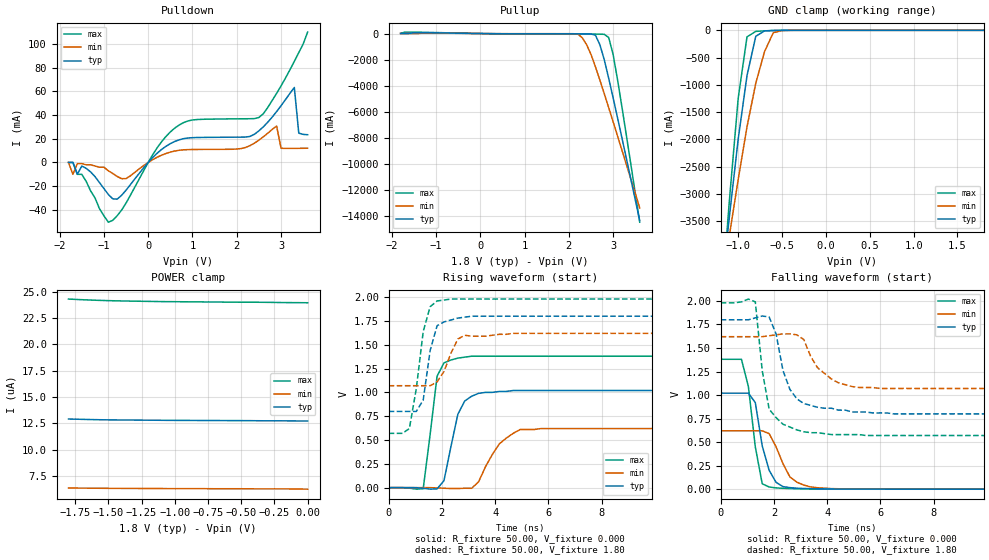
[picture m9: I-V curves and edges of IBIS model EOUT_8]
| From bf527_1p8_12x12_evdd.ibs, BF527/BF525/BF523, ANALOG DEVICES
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|   Model prwd0408swcdg_25
[Model]   EOUT_8
Model_type   I/O
Polarity   Non-Inverting
Enable   Active-Low
Vinl =   0.70V
Vinh =   1.00V
Vmeas =   1.20V
Cref =  50.00pF
Rref =   1.00M
Vref =  0.000V
C_comp   4.57pF   4.11pF   5.03pF
[Temperature Range]   25.00   0.12k   -40.00
[Voltage Range]   1.80V   1.62V   1.98V
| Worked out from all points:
|   slope of the pulldown table from 0 to 0.27 V, typ, clamps not added: 27.1 ohm
|   slope of the pullup table from 0 to 0.27 V, typ, clamps not added: 27 ohm
|   GND clamp passes 1 mA (typ) near -0.53 V on its own axis
|   rising waveform, R_fixture 50.00, V_fixture 0.000: 20-80 % time 510ps typ, 833ps min, 361ps max; typ from 0 V to 1.02 V
|   rising waveform, R_fixture 50.00, V_fixture 1.80: 20-80 % time 380ps typ, 528ps min, 434ps max; typ from 0.8 V to 1.8 V
|   falling waveform, R_fixture 50.00, V_fixture 0.000: 20-80 % time 457ps typ, 633ps min, 388ps max; typ from 1.02 V to 0 V
|   falling waveform, R_fixture 50.00, V_fixture 1.80: 20-80 % time 643ps typ, 881ps min, 415ps max; typ from 1.8 V to 0.8 V
[Pulldown]
| voltage   I(typ)   I(min)   I(max)
-1.8V     0A         0A         0A
-1.7V     0A         -10mA      0A
-1.6V     -10mA      -1mA       -10mA
-1.4V     -5mA       -2mA       -16mA
-800mV    -30.7mA    -9.3mA     -48.84mA
500mV     15.88mA    8.74mA     25.75mA
2.5V      26.68mA    18.82mA    37.97mA
2.9V      42.93mA    30.68mA    58.3mA
3V        47.87mA    11.96mA    64.59mA
3.3V      63.26mA    11.89mA    85.33mA
3.4V      24.7mA     11.92mA    92.67mA
3.6V      23.41mA    12.01mA    110mA
[Pullup]
| voltage   I(typ)   I(min)   I(max)
-1.8V     1.57mA     550uA      11.24mA
-1.6V     3.17mA     560uA      110mA
2.2V      -22.72mA   -39.81mA   -37.76mA
2.3V      -23.19mA   -310mA     -37.83mA
2.4V      -25.42mA   -850mA     -37.96mA
2.6V      -130mA     -2.54A     -42.68mA
2.7V      -850mA     -3.56A     -49.75mA
2.8V      -2.01A     -4.61A     -61.07mA
2.9V      -3.43A     -5.68A     -310mA
3V        -4.93A     -6.76A     -1.61A
3.1V      -6.46A     -7.85A     -3.55A
3.6V      -14.31A    -13.35A    -14.44A
[GND_clamp]
| voltage   I(typ)   I(min)   I(max)
-1.8V     -14.28A    -11.35A    -18.41A
-1.2V     -4.9A      -4.81A     -5.19A
-1.1V     -3.4A      -3.75A     -3.1A
-1V       -1.99A     -2.73A     -1.24A
-900mV    -830mA     -1.77A     -120mA
-800mV    -110mA     -970mA     -19.23mA
-700mV    -9.9mA     -390mA     -9.79mA
-600mV    -2.58mA    -42.87mA   -3.52mA
-500mV    -470uA     -4.39mA    -570uA
1.8V      12.72uA    6.27uA     23.92uA
[POWER_clamp]
| voltage   I(typ)   I(min)   I(max)
-1.8V     12.91uA    6.36uA     24.3uA
-1.7V     12.88uA    6.35uA     24.24uA
-1.6V     12.85uA    6.34uA     24.19uA
-1.5V     12.83uA    6.33uA     24.15uA
-1.4V     12.82uA    6.32uA     24.12uA
-1.1V     12.79uA    6.31uA     24.06uA
-1V       12.78uA    6.3uA      24.05uA
-500mV    12.76uA    6.29uA     24uA
-400mV    12.75uA    6.28uA     24uA
-300mV    12.74uA    6.28uA     23.99uA
-200mV    12.74uA    6.28uA     23.97uA
0V        12.72uA    6.25uA     23.95uA
[Ramp]
| variable   typ   min   max
dV/dt_r   0.61/0.47n   0.37/0.71n   0.83/0.29n
dV/dt_f   0.60/0.64n   0.33/0.77n   0.84/0.40n
R_load = 50.00
[Rising Waveform]
R_fixture = 50.00
V_fixture = 0.000
V_fixture_min = 0.000
V_fixture_max = 0.000
L_fixture = 0.000H
C_fixture = 0.000F
| time   V(typ)   V(min)   V(max)
0s        0V         0V         0V
1.3ns     -7.2mV     43.91uV    -11.18mV
1.82ns    -13.54mV   -3.09mV    1.17V
2.08ns    73.34mV    -6.38mV    1.31V
2.34ns    430mV      -9.68mV    1.34V
2.86ns    910mV      -6.49mV    1.37V
3.38ns    990mV      61.21mV    1.38V
4.16ns    1.01V      460mV      1.38V
4.94ns    1.02V      610mV      1.38V
13ns      1.02V      620mV      1.38V
[Rising Waveform]
R_fixture = 50.00
V_fixture = 1.80
V_fixture_min = 1.62
V_fixture_max = 1.98
L_fixture = 0.000H
C_fixture = 0.000F
| time   V(typ)   V(min)   V(max)
0s        800mV      1.07V      570mV
780ps     800mV      1.07V      620mV
1.04ns    800mV      1.07V      1.04V
1.3ns     920mV      1.07V      1.64V
1.56ns    1.44V      1.07V      1.9V
1.82ns    1.7V       1.11V      1.96V
2.08ns    1.74V      1.22V      1.97V
2.6ns     1.78V      1.56V      1.98V
2.86ns    1.79V      1.6V       1.98V
13ns      1.8V       1.62V      1.98V
[Falling Waveform]
R_fixture = 50.00
V_fixture = 0.000
V_fixture_min = 0.000
V_fixture_max = 0.000
L_fixture = 0.000H
C_fixture = 0.000F
| time   V(typ)   V(min)   V(max)
0s        1.02V      620mV      1.38V
780ps     1.02V      620mV      1.38V
1.04ns    1.02V      620mV      1.09V
1.3ns     920mV      620mV      450mV
1.56ns    460mV      620mV      57.34mV
1.82ns    200mV      590mV      23.02mV
2.08ns    72.55mV    450mV      13.37mV
2.6ns     16.19mV    130mV      6.68mV
3.38ns    5.63mV     23.46mV    2.15mV
13ns      -24.56uV   9.5uV      -30.31uV
[Falling Waveform]
R_fixture = 50.00
V_fixture = 1.80
V_fixture_min = 1.62
V_fixture_max = 1.98
L_fixture = 0.000H
C_fixture = 0.000F
| time   V(typ)   V(min)   V(max)
0s        1.8V       1.62V      1.98V
1.3ns     1.82V      1.62V      1.99V
1.56ns    1.84V      1.62V      1.26V
1.82ns    1.83V      1.63V      850mV
2.08ns    1.65V      1.64V      760mV
2.34ns    1.26V      1.65V      690mV
2.86ns    960mV      1.64V      630mV
3.64ns    870mV      1.29V      600mV
4.94ns    820mV      1.09V      580mV
13ns      800mV      1.07V      570mV
